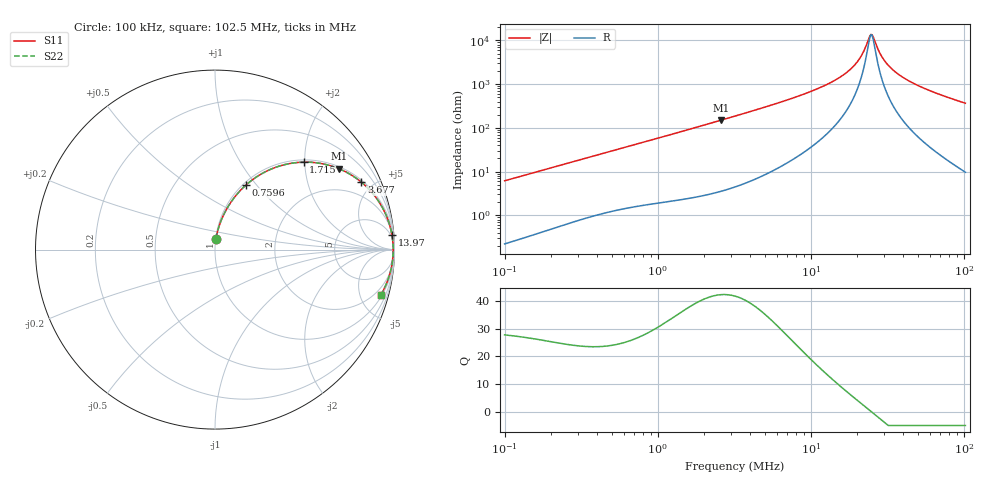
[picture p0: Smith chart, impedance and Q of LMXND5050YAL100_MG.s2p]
! LMXND5050YAL100_MG  S-PARAMETER MODEL  ( General Type )
! Model Generated by TAIYO YUDEN Corporation (http://www.ty-top.com)
! Version 1.0
! TAIYO YUDEN Control No. 191023NI43SB-FBB
! Copyright(c) 2019 TAIYO YUDEN CO.,LTD. All Rights Reserved.
! Product Description (link to TY-COMPAS)
! https://ds.yuden.co.jp/TYCOMPAS/or/detail?pn=LMXND5050YAL100MMG&u=M
! Products Name : Inductors
! Characteristics :
!  Inductance : 10 uH , SRF(min) : 18 MHz , DC Resistance(max) : 0.0728 Ohm
!  Rated Current : Saturation :2300 mA , Temp Rise : 2100 mA
!  Case Size : 4.9 x 4.9 / 0.193 x 0.193 [mm/inch] , Thickness : 4.1 / 0.161 [mm/inch]
!  (Conditions: Temperature = 25 degC , DC Bias Current/Voltage = 0A / 0V)
! External Node Assignments :
!  1  o---GGG---o  2
! GND o---------o GND
! Frequency Range : 0.1MHz  -  102.47202MHz  [ 402 STEP ]
# MHz S RI R 50
! Freq[MHz].  S11 Real  S11 Imag  S21 Real  S21 Imag  S12 Real  S12 Imag  S22 Real  S22 Imag
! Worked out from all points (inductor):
!   401 points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, 100 kHz to 102.5 MHz, reference 50 ohm
!   read as one part in series: L = 9.74 uH near 103.5 kHz
!   highest Q = 42.4 at 2.6 MHz (marker M1), where L = 9.2 uH
!   self-resonance near 24.74 MHz
!   S11 on the Smith chart (normalised r, x): 100 kHz: 1.00, +0.12; 759.6 kHz: 1.03, +0.88; 1.715 MHz: 1.05, +1.98; 3.677 MHz: 1.11, +4.30; 13.97 MHz: 3, +23; 102.5 MHz: 1.19, -7.33
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0.1  0.00595 0.061  0.994 -0.061  0.994 -0.061  0.00595 0.061
0.319357  0.0424 0.1814  0.9576 -0.1814  0.9576 -0.1814  0.0424 0.1814
0.75963  0.1725 0.3598  0.8275 -0.3598  0.8275 -0.3598  0.1725 0.3598
1.019889  0.2649 0.4254  0.7351 -0.4254  0.7351 -0.4254  0.2649 0.4254
1.715332  0.4944 0.4873  0.5056 -0.4873  0.5056 -0.4873  0.4944 0.4873
2.600067  0.6893 0.4511  0.3107 -0.4511  0.3107 -0.4511  0.6893 0.4511
3.257086  0.7766 0.4047  0.2234 -0.4047  0.2234 -0.4047  0.7766 0.4047
3.677179  0.8159 0.3754  0.1841 -0.3754  0.1841 -0.3754  0.8159 0.3754
5.770376  0.9169 0.2609  0.0831 -0.2609  0.0831 -0.2609  0.9169 0.2609
10.22302  0.9729 0.1375  0.0271 -0.1375  0.0271 -0.1375  0.9729 0.1375
13.96549  0.9854 0.084  0.0146 -0.084  0.0146 -0.084  0.9854 0.084
16.89849  0.9897 0.0549  0.0103 -0.0549  0.0103 -0.0549  0.9897 0.0549
19.75088  0.9917 0.0323  0.00829 -0.0323  0.00829 -0.0323  0.9917 0.0323
21.53868  0.9924 0.0201  0.00762 -0.0201  0.00762 -0.0201  0.9924 0.0201
23.89891  0.9928 0.00563  0.00722 -0.00563  0.00722 -0.00563  0.9928 0.00563
24.74179  0.9928 0.000816  0.00719 -0.000816  0.00719 -0.000816  0.9928 0.000816
25.6144  0.9928 -0.00399  0.0072 0.00399  0.0072 0.00399  0.9928 -0.00399
29.42364  0.9923 -0.0233  0.00771 0.0233  0.00771 0.0233  0.9923 -0.0233
32.64791  0.9914 -0.0381  0.00861 0.0381  0.00861 0.0381  0.9914 -0.0381
38.82581  0.9888 -0.0635  0.0112 0.0635  0.0112 0.0635  0.9888 -0.0635
49.48707  0.9823 -0.1019  0.0177 0.1019  0.0177 0.1019  0.9823 -0.1019
102.472  0.9251 -0.2504  0.0749 0.2504  0.0749 0.2504  0.9251 -0.2504
